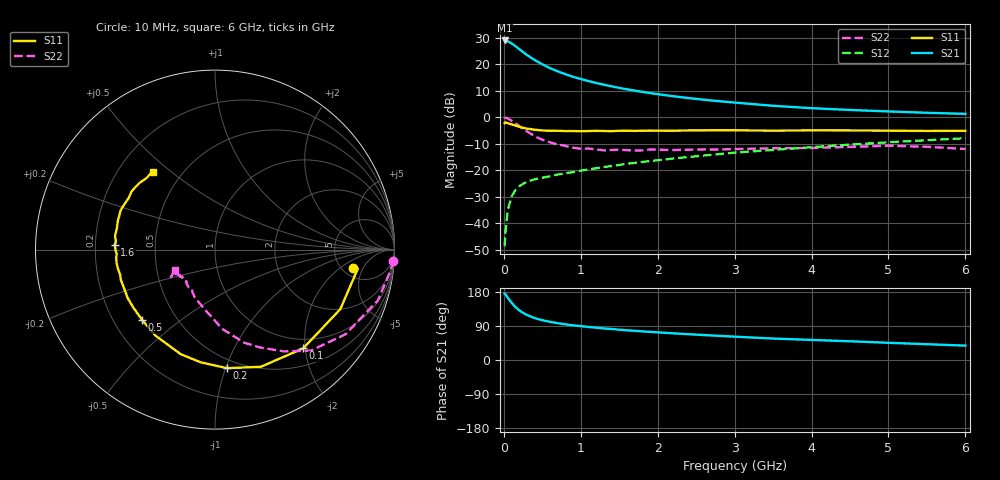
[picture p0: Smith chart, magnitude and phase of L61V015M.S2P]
!  INFINEON TECHNOLOGIES Small Signal Semiconductors
! BFR380L3 , Si-NPN RF-Transistor in TSLP-3-1
!  Vce=1 V,  Ic=15 mA
! Common Emitter S-Parameters:  07. March 2005
#  GHz  S  MA  R  50
! f  S11  S21  S12  S22
! GHz  Mag  Ang  Mag  Ang  Mag  Ang  Mag  Ang
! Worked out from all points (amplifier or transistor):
!   36 points, 10 MHz to 6 GHz, reference 50 ohm
!   highest |S21| = 29.0 dB at 10 MHz (marker M1)
!   |S21| within 3 dB of that: start of sweep to 188.5 MHz
!   unconditionally stable (mu >= 1): 1.935 GHz to 4.998 GHz
!   at 250 MHz: K = 0.32, MSG = 24.9 dB, |S12| = -25.1 dB
!   at 1.4 GHz: K = 0.94, MSG = 15.0 dB, |S12| = -18.4 dB
!   at 6 GHz: K = 0.99, MSG = 4.6 dB, |S12| = -7.9 dB
!   S11 on the Smith chart (normalised r, x): 10 MHz: 6.26, -3.26; 100 MHz: 0.81, -1.96; 200 MHz: 0.43, -1.01; 500 MHz: 0.32, -0.37; 1.6 GHz: 0.28, +0.02; 6 GHz: 0.34, +0.43
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0.01  0.7775 -7.6  28.19 175.1  0.0037 80.0  0.9961 -3.6
0.02  0.8025 -7.7  27.95 174.0  0.0065 84.0  0.9832 -7.2
0.05  0.773 -25.4  27.25 164.6  0.0173 79.3  0.9507 -17.3
0.1  0.7378 -48.2  24.86 151.1  0.032 68.2  0.8672 -32.9
0.15  0.7011 -68.6  22.09 139.8  0.0423 60.4  0.776 -46.5
0.2  0.6641 -84.2  19.36 131.1  0.05 55.3  0.684 -56.0
0.25  0.633 -97.2  17.04 124.4  0.0557 51.2  0.5995 -65.4
0.3  0.6131 -108.2  15.01 118.8  0.0607 49.1  0.5432 -72.6
0.4  0.5828 -124.7  12.07 110.6  0.0674 46.6  0.4422 -85.0
0.5  0.5643 -136.0  10.01 105.1  0.0725 46.5  0.3768 -92.6
0.6  0.558 -144.9  8.46 100.6  0.077 46.8  0.3372 -100.1
0.8  0.5503 -157.3  6.507 94.1  0.0876 48.9  0.2885 -113.2
0.9  0.5511 -162.3  5.81 91.6  0.0924 50.5  0.2677 -118.1
1.1  0.5512 -169.0  4.824 87.2  0.1039 52.7  0.257 -124.4
1.3  0.5517 -175.5  4.127 83.3  0.1156 54.2  0.2376 -132.2
1.6  0.5597 177.2  3.376 78.4  0.1326 56.3  0.2399 -139.6
2.2  0.5598 166.8  2.501 70.4  0.1668 58.5  0.2414 -143.4
2.8  0.5695 157.7  2.011 63.7  0.2019 59.9  0.2475 -149.2
3.5  0.5603 148.9  1.648 56.6  0.2424 58.9  0.2602 -148.8
4.5  0.5648 142.3  1.376 49.4  0.3053 58.2  0.276 -148.7
5.5  0.5521 133.8  1.217 41.7  0.3695 54.9  0.2779 -149.3
6  0.5564 128.6  1.16 37.9  0.4029 53.0  0.2523 -152.9
